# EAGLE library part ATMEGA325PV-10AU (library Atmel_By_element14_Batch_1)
8-bit Microcontroller with 32K Bytes In-System Programmable Programmable
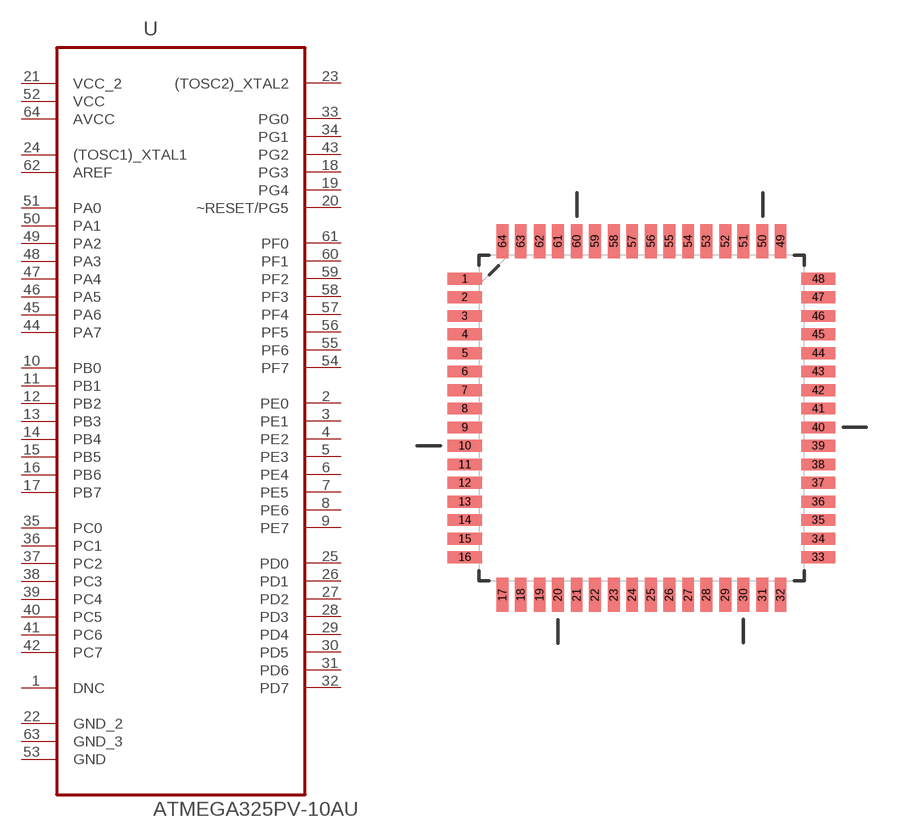
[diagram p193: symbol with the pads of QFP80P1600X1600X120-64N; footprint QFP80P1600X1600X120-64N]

Designator prefix U

## ATMEGA325PV-10AU (MPN: ATMEGA325PV-10AU; OC_FARNELL: 1636940; OC_NEWARK: 03P2025; PACKAGE: TQFP-64; SUPPLIER: Atmel)  [QFP80P1600X1600X120-64N]
1  DNC  nc
2  PE0
3  PE1
4  PE2
5  PE3
6  PE4
7  PE5
8  PE6
9  PE7
10  PB0
11  PB1
12  PB2
13  PB3
14  PB4
15  PB5
16  PB6
17  PB7
18  PG3
19  PG4
20  ~RESET/PG5
21  VCC_2  pwr
22  GND_2  pas
23  (TOSC2)_XTAL2  out
24  (TOSC1)_XTAL1  in
25  PD0
26  PD1
27  PD2
28  PD3
29  PD4
30  PD5
31  PD6
32  PD7
33  PG0
34  PG1
35  PC0
36  PC1
37  PC2
38  PC3
39  PC4
40  PC5
41  PC6
42  PC7
43  PG2
44  PA7
45  PA6
46  PA5
47  PA4
48  PA3
49  PA2
50  PA1
51  PA0
52  VCC  pwr
53  GND  pas
54  PF7
55  PF6
56  PF5
57  PF4
58  PF3
59  PF2
60  PF1
61  PF0
62  AREF  in
63  GND_3  pas
64  AVCC  pwr

## Footprint QFP80P1600X1600X120-64N (pad centres in mm)
smd 1.473 x 0.508: 1 -7.62,5.994; 2 -7.62,5.207; 3 -7.62,4.394; 4 -7.62,3.607; 5 -7.62,2.794; 6 -7.62,2.007; 7 -7.62,1.194; 8 -7.62,0.406; 9 -7.62,-0.406; 10 -7.62,-1.194; 11 -7.62,-2.007; 12 -7.62,-2.794; 13 -7.62,-3.607; 14 -7.62,-4.394; 15 -7.62,-5.207; 16 -7.62,-5.994; 33 7.62,-5.994; 34 7.62,-5.207; 35 7.62,-4.394; 36 7.62,-3.607; 37 7.62,-2.794; 38 7.62,-2.007; 39 7.62,-1.194; 40 7.62,-0.406; 41 7.62,0.406; 42 7.62,1.194; 43 7.62,2.007; 44 7.62,2.794; 45 7.62,3.607; 46 7.62,4.394; 47 7.62,5.207; 48 7.62,5.994
smd 0.508 x 1.473: 17 -5.994,-7.62; 18 -5.207,-7.62; 19 -4.394,-7.62; 20 -3.607,-7.62; 21 -2.794,-7.62; 22 -2.007,-7.62; 23 -1.194,-7.62; 24 -0.406,-7.62; 25 0.406,-7.62; 26 1.194,-7.62; 27 2.007,-7.62; 28 2.794,-7.62; 29 3.607,-7.62; 30 4.394,-7.62; 31 5.207,-7.62; 32 5.994,-7.62; 49 5.994,7.62; 50 5.207,7.62; 51 4.394,7.62; 52 3.607,7.62; 53 2.794,7.62; 54 2.007,7.62; 55 1.194,7.62; 56 0.406,7.62; 57 -0.406,7.62; 58 -1.194,7.62; 59 -2.007,7.62; 60 -2.794,7.62; 61 -3.607,7.62; 62 -4.394,7.62; 63 -5.207,7.62; 64 -5.994,7.62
